| PGE_DESIGN_SPEC   IBIS MODEL
[IBIS Ver]   3.2
[File Name]   sprm479.ibs
[File Rev]   1.00
[Date]   Feb 3, 2003
[Source]   Data created at ZUKEN
[Notes]   File originated from TISPICE Simulation.
|   Feb 3, 2003 : First release
|   Notes:
|   -Some IV curves contain Non monotonic data points. They are
|   appropriate calculation results.
|   -Extreme current warnings are not the problem. The currents
|   correspond to the results of SPICE simulation.
|   -The warnings of 'value never becomes zero' are due to
|   IV curves which do not pass the zero voltage level. They are
|   not the problem, are caused by a voltage shift due to an
|   active resistor function.
|   -Some input cells do not have a power clamp diode. In this
|   case, current level in [POWER_Clamp] table is very low.
|   -This model contains a submodel definition. If your simulator
|   stops due to the errors, please follow instructions which
|   the simulator indicated, or remove the submodel section.
[Disclaimer]   Please be aware that in the absence of a written agreement
|   Texas Instruments(TI) assumes no liability for:
|   (1) The accuracy of the IBIS models provided to your company
|   (2) The proper functioning of these Models in your design
|   or for any resulting applications;or property rights
|   resulting from your use of these models. TI provides IBIS
|   Models as a service to our customers and therefore reserves
|   the right to limit distribution of the Models.
[Copyright]   Property of Texas Instruments Incorporated.
|   Unauthorised reproduction and/or distribution is strictly
|   prohibited. This product is protected under copyright law and
|   trade secret law as an unpublished work.
|   Created 2003,(C) Copyright 2003,
|   Texas Instruments Incorporated., All Rights Reserved.
| Component   C5509_PGE
[Component]   C5509_PGE
[Manufacturer]   Texas Instruments
[Package]
| Variable   Typ   Min   Max
R_pkg   0.1088   0.07437   0.1226
L_pkg   6.853e-09   6.184e-09   7.767e-09
C_pkg   1.256e-12   8.778e-13   1.487e-12
[Pin]  signal_name  model_name   R_pin   L_pin   C_pin
1   VSS   GND   0.0805   7.767e-09   1.237e-12
2   pu   OUI831   0.122   7.716e-09   1.487e-12
3   dp   UIS245_UIS246_UOS181  0.121   7.563e-09   1.423e-12
4   dn   UIS245_UIS246_UOS181  0.1226   7.499e-09   1.412e-12
5   VDDSHV2   POWER   0.1212   7.33e-09   1.409e-12
6   gpio7   IDG091_OUI831   0.1203   7.21e-09   1.316e-12
7   VSS   GND   0.07829   6.893e-09   1.313e-12
8   VDDSHV   POWER   0.07815   6.778e-09   1.362e-12
9   gpio2   IDG091_OUI831   0.1193   6.855e-09   1.314e-12
10   gpio1   IDG091_OUI831   0.1186   6.772e-09   1.231e-12
11   VSS   GND   0.07692   6.487e-09   1.244e-12
12   gpio0   IDG091_OUI831   0.1178   6.569e-09   1.239e-12
|13   x2clkin   UIS471   0.1168   6.474e-09   1.214e-12
|14   x1   UOS339   0.1164   6.42e-09   1.175e-12
15   clkout   OUKB31   0.1159   6.365e-09   1.159e-12
16   c0   OUI831_UPS239ON   0.1154   6.323e-09   1.147e-12
17   c1   OUI831   0.115   6.299e-09   1.115e-12
18   VDD   POWER   0.07437   6.184e-09   9.153e-13
19   c2   OUI831_UPS239ON   0.1166   6.277e-09   8.778e-13
20   c3   IDG091_OUI831   0.1162   6.31e-09   1.107e-12
21   c4   OUI831_UPS239ON   0.1157   6.327e-09   1.133e-12
22   c5   OUI831_UPS239ON   0.1152   6.356e-09   1.151e-12
23   c6   OUI831_UPS239ON   0.1155   6.403e-09   1.166e-12
24   VDDSHV   POWER   0.0744   6.245e-09   1.229e-12
25   c7   OUI831_UPS239ON   0.1155   6.519e-09   1.233e-12
26   c8   OUI831_UPS239ON   0.1161   6.628e-09   1.21e-12
27   c9   OUI831_UPS239ON   0.1158   6.709e-09   1.224e-12
28   c11   OUI831_UPS239ON   0.1161   6.787e-09   1.297e-12
29   VDD   POWER   0.1169   6.905e-09   1.326e-12
30   VDD   POWER   0.1178   7.054e-09   1.301e-12
31   c14   OUI831_UPS239ON   0.1188   7.198e-09   1.313e-12
32   c12   OUI831_UPS239ON   0.1182   7.265e-09   1.379e-12
33   VSS   GND   0.07745   7.176e-09   1.444e-12
34   c10   OUI831_UPS239ON   0.1197   7.555e-09   1.45e-12
35   c13   OUI831_UPS239ON   0.1204   7.731e-09   1.457e-12
36   VSS   GND   0.07892   7.741e-09   1.196e-12
37   VSS   GND   0.09156   8.062e-09   1.233e-12
38   a13   OUI831_UPS239ON   0.1407   8.062e-09   1.478e-12
39   a12   OUI831_UPS239ON   0.1405   7.936e-09   1.447e-12
40   a11   OUI831_UPS239ON   0.1392   7.771e-09   1.424e-12
41   VDD   POWER   0.08967   7.432e-09   1.437e-12
42   a10   OUI831_UPS239ON   0.1392   7.581e-09   1.343e-12
43   a9   OUI831_UPS239ON   0.1384   7.463e-09   1.319e-12
44   a8   OUI831_UPS239ON   0.1375   7.329e-09   1.34e-12
45   VSS   GND   0.08827   7.016e-09   1.346e-12
46   a7   OUI831_UPS239ON   0.1375   7.176e-09   1.259e-12
47   a6   OUI831_UPS239ON   0.1376   7.102e-09   1.239e-12
48   a5   OUI831_UPS239ON   0.1369   7.001e-09   1.251e-12
49   VDDSHV   POWER   0.08694   6.691e-09   1.268e-12
50   a4   OUI831_UPS239ON   0.1365   6.875e-09   1.212e-12
51   a3   OUI831_UPS239ON   0.136   6.835e-09   1.189e-12
52   a2   OUI831_UPS239ON   0.1356   6.799e-09   1.173e-12
53   VDD   POWER   0.08587   6.542e-09   1.167e-12
54   a1   OUI831_UPS239ON   0.1367   6.869e-09   9.351e-13
55   a0   OUI831_UPS239ON   0.1387   6.766e-09   9.02e-13
56   VDDSHV   POWER   0.08702   6.549e-09   1.164e-12
57   d0   OUI831_UPS239ON   0.1373   6.809e-09   1.178e-12
58   d1   OUI831_UPS239ON   0.1375   6.849e-09   1.189e-12
59   d2   OUI831_UPS239ON   0.1377   6.897e-09   1.199e-12
60   VSS   GND   0.08726   6.697e-09   1.268e-12
61   d3   OUI831_UPS239ON   0.1379   7.017e-09   1.267e-12
62   d4   OUI831_UPS239ON   0.1384   7.123e-09   1.248e-12
63   d5   OUI831_UPS239ON   0.1391   7.226e-09   1.258e-12
64   VSS   GND   0.08878   7.046e-09   1.351e-12
65   d6   OUI831_UPS239ON   0.1391   7.386e-09   1.35e-12
66   d7   OUI831_UPS239ON   0.1383   7.479e-09   1.31e-12
67   d8   OUI831_UPS239ON   0.1389   7.6e-09   1.329e-12
68   VDD   POWER   0.08884   7.414e-09   1.436e-12
69   d9   OUI831_UPS239ON   0.1386   7.782e-09   1.443e-12
70   d10   OUI831_UPS239ON   0.1399   7.959e-09   1.455e-12
71   d11   OUI831_UPS239ON   0.1405   8.11e-09   1.47e-12
72   VDDSHV   POWER   0.09088   8.083e-09   1.213e-12
73   VSS   GND   0.1224   7.963e-09   1.162e-12
74   d12   OUI831_UPS239ON   0.1235   7.793e-09   1.454e-12
75   d13   OUI831_UPS239ON   0.1224   7.619e-09   1.451e-12
76   d14   OUI831_UPS239ON   0.1206   7.427e-09   1.415e-12
77   d15   OUI831_UPS239ON   0.1207   7.313e-09   1.382e-12
78   VDD   POWER   0.0789   7.026e-09   1.351e-12
79   emu0   IDG041OUI831PS1001ON  0.1199   7.085e-09   1.316e-12
80   emu1   IDG041OUI831PS1001ON  0.1187   6.939e-09   1.331e-12
81   tdo   OUI831   0.1177   6.817e-09   1.301e-12
82   tdi   IDG041_PS1001ON   0.1171   6.733e-09   1.227e-12
83   VDD   POWER   0.07609   6.453e-09   1.239e-12
84   trstn   IDG041_PE1001ON   0.1164   6.536e-09   1.236e-12
85   tck   IDG091_PS1001ON   0.1155   6.446e-09   1.211e-12
86   tms   IDG041_PS1001ON   0.1152   6.399e-09   1.161e-12
87   VDD   POWER   0.07512   6.176e-09   1.161e-12
88   VDDSHV   POWER   0.07525   6.141e-09   1.171e-12
89   sda   IDI091_UOS205   0.1165   6.306e-09   1.127e-12
90   scl   IDI091_UOS205   0.1165   6.388e-09   9.093e-13
91   nreset   IDG091   0.1168   6.278e-09   8.724e-13
92   VSS   GND   0.1157   6.306e-09   1.11e-12
93   nint0   IDG091   0.1159   6.328e-09   1.147e-12
94   nint1   IDG091   0.1162   6.369e-09   1.159e-12
95   VDD   POWER   0.1165   6.423e-09   1.167e-12
96   nint2   IDG091   0.1158   6.456e-09   1.204e-12
97   nint3   IDG091   0.1165   6.549e-09   1.222e-12
98   VDDSHV   POWER   0.07568   6.442e-09   1.238e-12
99   nint4   IDG091   0.1169   6.733e-09   1.241e-12
100   VSS   GND   0.1173   6.822e-09   1.3e-12
101   xf   OUI831   0.1181   6.945e-09   1.329e-12
102   VSS   GND   0.1191   7.097e-09   1.297e-12
103   VSS3V   GND   0.07783   7e-09   1.347e-12
104   VDD3VHV   POWER   0.1195   7.308e-09   1.412e-12
|105   ain0   SW0101   0.1207   7.48e-09   1.429e-12
|106   ain1   SW0101   0.1223   7.677e-09   1.434e-12
107   VDDAHV   POWER   0.1205   7.737e-09   1.437e-12
108   VSSA   GND   0.07893   7.742e-09   1.195e-12
109   VDD5   POWER   0.09178   8.076e-09   1.233e-12
110   VDD4   POWER   0.1412   8.079e-09   1.474e-12
|111   rtcx2   OS11V1   0.1415   7.974e-09   1.437e-12
|112   rtcx1   OS11H1   0.1412   7.845e-09   1.419e-12
113   VSS   GND   0.1416   7.748e-09   1.411e-12
114   VSS   GND   0.1411   7.647e-09   1.343e-12
115   VSS   GND   0.1401   7.516e-09   1.324e-12
116   s23   OUI831_UPS239ON   0.1392   7.378e-09   1.35e-12
117   s25   IDG041_OUI831   0.1386   7.269e-09   1.315e-12
118   VDD   POWER   0.0891   6.989e-09   1.283e-12
119   s24   IDG091_OUI831   0.1387   7.119e-09   1.252e-12
120   s21   IDG041_OUI831   0.1381   7.026e-09   1.248e-12
121   s22   IDG041_OUI831   0.1384   6.959e-09   1.232e-12
122   VSS   GND   0.1382   6.91e-09   1.204e-12
123   s20   IDG091_OUI831   0.1376   6.855e-09   1.191e-12
124   s13   OUI831_UPS239ON   0.1371   6.814e-09   1.179e-12
125   s15   IDG041_OUI831   0.1367   6.791e-09   1.146e-12
126   VDDSHV1   POWER   0.1375   6.876e-09   9.292e-13
127   s14   IDG091_OUI831   0.1388   6.768e-09   9.141e-13
128   s11   IDG041_OUI831   0.1392   6.81e-09   1.146e-12
129   s12   IDG041_OUI831   0.1388   6.831e-09   1.165e-12
130   s10   IDG091_OUI831   0.138   6.859e-09   1.181e-12
131   dx0   OUI831   0.1382   6.907e-09   1.197e-12
132   VDD   POWER   0.0874   6.702e-09   1.262e-12
133   fsx0   IDG041_OUI831   0.1379   7.018e-09   1.262e-12
134   clkx0   IDG091_OUI831   0.1383   7.121e-09   1.246e-12
135   dr0   IDG041   0.1389   7.222e-09   1.261e-12
136   fsr0   IDG041_OUI831   0.1391   7.295e-09   1.325e-12
137   clkr0   IDG091_OUI831   0.1396   7.403e-09   1.348e-12
138   VSS   GND   0.08964   7.278e-09   1.341e-12
139   VDDSHV1   POWER   0.08968   7.374e-09   1.351e-12
140   tinout0   IDG091_OUI831   0.1373   7.63e-09   1.402e-12
141   gpio6   IDG091_OUI831   0.1382   7.775e-09   1.427e-12
142   gpio4   IDG091_OUI831   0.1384   7.906e-09   1.443e-12
143   gpio3   IDG091_OUI831   0.139   8.054e-09   1.466e-12
144   VSS   GND   0.09014   8.032e-09   1.208e-12
[Diff Pin] inv_pin   vdiff   tdelay_typ   tdelay_min   tdelay_max
3   4   0.2   NA   NA   NA
| Models and submodels in the file (14): OUI831 (3-state), OUKB31 (3-state), IDG091 (Input), IDG041 (Input), IDG041_PS1001ON (Input), IDG091_PS1001ON (Input), IDG041_PE1001ON (Input), IDI091_UOS205 (I/O_open_drain), IDG041OUI831PS1001ON (I/O), IDG091_OUI831 (I/O), OUI831_UPS239ON (I/O), UPS239BH (Bus_hold), IDG041_OUI831 (I/O), UIS245_UIS246_UOS181 (I/O)
